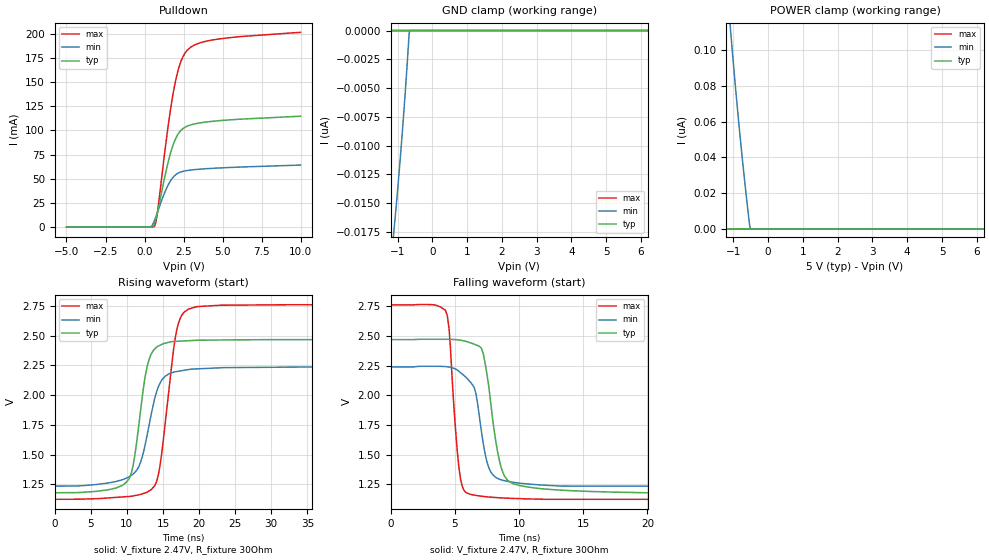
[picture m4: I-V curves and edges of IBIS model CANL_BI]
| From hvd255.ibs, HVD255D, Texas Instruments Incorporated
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[Model]   CANL_BI
Model_type   I/O_open_drain
Polarity   Non-Inverting
Vinl = 0.5V
Vinh = 0.9V
Vmeas = 2.47V
Vref = 2.47V
Rref = 30
|   typ   min   max
|   (nom PVT)   (slow PVT)   (fast PVT)
C_comp   13.675pF   13.224pF   13.735pF
|C_comp (Dom state)   13.675pF   13.224pF   13.735pF
|   (nom PVT)   (fast PVT)   (slow PVT)
|C_comp (Rec state)   4.9637pF   3.1317pF   7.3060pF
[Voltage Range]   5   4.5   5.5
[Temperature Range]   27   125   -40
[Pullup Reference]   5   4.5   5.5
[Pulldown Reference]   -0   -0   -0
[Power Clamp Reference]   5   4.5   5.5
[GND Clamp Reference]   -0   -0   -0
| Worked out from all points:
|   slope of the pulldown table from 0 to 0.75 V, typ, clamps not added: 77.8 ohm
|   falling waveform, V_fixture 2.47V, R_fixture 30Ohm: 20-80 % time 1.06ns typ, 935ps min, 627ps max; typ from 2.47 V to 1.18 V
|   rising waveform, V_fixture 2.47V, R_fixture 30Ohm: 20-80 % time 1.76ns typ, 2.29ns min, 1.89ns max; typ from 1.18 V to 2.47 V
[Pulldown]
|   Voltage   I(typ)   I(min)   I(max)
-5V       -1.176pA   -6.038pA   -931.4fA
265mV     448.6nA    26.14uA    19.87nA
460mV     72.13uA    1.2mA      2.383uA
625mV     2.868mA    6.415mA    697.1uA
805mV     13.43mA    14.38mA    12.94mA
1.48V     65.21mA    42.6mA     100.9mA
1.9V      87.96mA    52.76mA    144.1mA
2.095V    94.72mA    55.26mA    158.7mA
2.35V     100.3mA    57.12mA    172.1mA
2.935V    105.5mA    58.95mA    185.6mA
4.825V    110mA      61.16mA    194.5mA
9.985V    114.6mA    64.11mA    201.2mA
[GND Clamp]
|   Voltage   I(typ)   I(min)   I(max)
-5V       -1.547nA   -139.9nA   -1.04nA
-4.97V    0A         -72.79nA   0A
-1.1V     0A         -17.31nA   0A
-1.07V    0A         -16.34nA   0A
-980mV    0A         -13.27nA   0A
-875mV    0A         -9.366nA   0A
-815mV    0A         -6.953nA   0A
-770mV    0A         -5.046nA   0A
-710mV    0A         -2.359nA   0A
-665mV    0A         -225.3pA   0A
-635mV    0A         0A         0A
9.985V    0A         0A         0A
[POWER Clamp]
|   Voltage   I(typ)   I(min)   I(max)
-5V       23.97nA    1.609uA    39.78nA
-4.97V    0A         1.483uA    0A
-1.085V   0A         112.9nA    0A
-1.055V   0A         105.8nA    0A
-965mV    0A         85.39nA    0A
-890mV    0A         69.25nA    0A
-815mV    0A         53.89nA    0A
-740mV    0A         39.28nA    0A
-635mV    0A         19.99nA    0A
-530mV    0A         1.983nA    0A
-500mV    0A         0A         0A
9.985V    0A         0A         0A
[Ramp]
R_load = 30
|   typ   min   max
dV/dt_r   0.775002/1.76232e-09   0.603473/2.27983e-09   0.983918/1.89162e-09
dV/dt_f   0.775237/1.05562e-09   0.6038/9.34833e-10   0.98411/6.26669e-10
[Falling Waveform]
V_fixture = 2.47V
V_fixture_min = 2.24V
V_fixture_max = 2.763V
R_fixture = 30Ohm
C_fixture = 0F
|   Time   V(typ)   V(min)   V(max)
0s        2.47V      2.24V      2.763V
4.28ns    2.473V     2.242V     2.716V
4.56ns    2.472V     2.238V     2.556V
5.449ns   2.465V     2.191V     1.293V
6.52ns    2.431V     2.063V     1.159V
7.384ns   2.255V     1.496V     1.145V
8.2ns     1.607V     1.308V     1.138V
8.9ns     1.314V     1.279V     1.134V
12.54ns   1.205V     1.239V     1.123V
139.9ns   1.178V     1.234V     1.123V
[Rising Waveform]
V_fixture = 2.47V
V_fixture_min = 2.24V
V_fixture_max = 2.763V
R_fixture = 30Ohm
C_fixture = 0F
|   Time   V(typ)   V(min)   V(max)
0s        1.178V     1.234V     1.123V
10.16ns   1.284V     1.308V     1.146V
10.86ns   1.409V     1.336V     1.151V
11.84ns   1.845V     1.426V     1.163V
12.82ns   2.244V     1.669V     1.184V
13.78ns   2.384V     1.954V     1.232V
14.62ns   2.421V     2.104V     1.421V
17ns      2.453V     2.199V     2.572V
19.6ns    2.461V     2.221V     2.743V
139.9ns   2.47V      2.239V     2.763V
